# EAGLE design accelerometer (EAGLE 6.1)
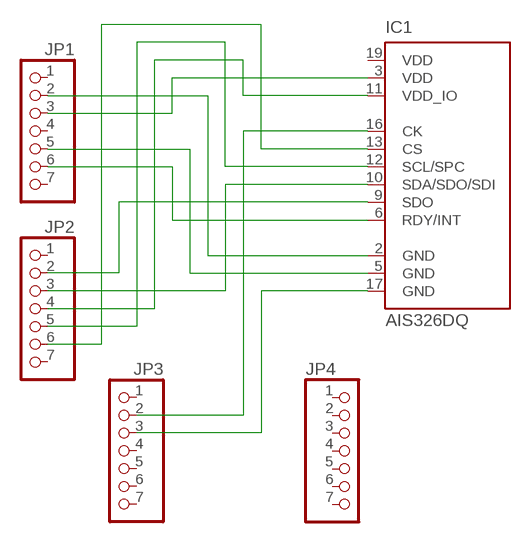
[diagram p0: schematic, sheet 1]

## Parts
IC1  AIS326DQ  [QFPN-28]
JP1  PINHD-1X7  [1X07]
JP2  PINHD-1X7  [1X07]
JP3  PINHD-1X7  [1X07]
JP4  PINHD-1X7  [1X07]

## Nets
N$1: IC1.2(GND) JP1.2
N$2: IC1.3(VDD) JP1.3
N$3: IC1.5(GND) JP1.5
N$4: IC1.6(RDY/INT) JP1.6
N$5: IC1.9(SDO) JP2.2
N$6: IC1.10(SDA/SDO/SDI) JP2.3
N$7: IC1.11(VDD_IO) JP2.4
N$8: IC1.12(SCL/SPC) JP2.5
N$9: IC1.13(CS) JP2.6
N$10: IC1.16(CK) JP3.2
N$11: IC1.17(GND) JP3.3
Unconnected: JP1.1 JP1.4 JP1.7 JP2.1 JP2.7 JP3.1 JP3.4 JP3.5 JP3.6 JP3.7 JP4.1 JP4.2 JP4.3 JP4.4 JP4.5 JP4.6 JP4.7

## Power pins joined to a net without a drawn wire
VDD: IC1.19(VDD)

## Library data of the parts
IC1 = cansat_jecnaci:AIS326DQ: MEMS INERTIAL SENSOR 3-Axis - ±2g/±6g Digital Output Low Voltage Linear Accelerometer Source: http://www.st.com; MF: Arrow Electronics; MPN: AIS326DQ; OC_FARNELL: 1220909; OC_NEWARK: 89K0642
JP1-JP4 = pinhead:PINHD-1X7: PIN HEADER

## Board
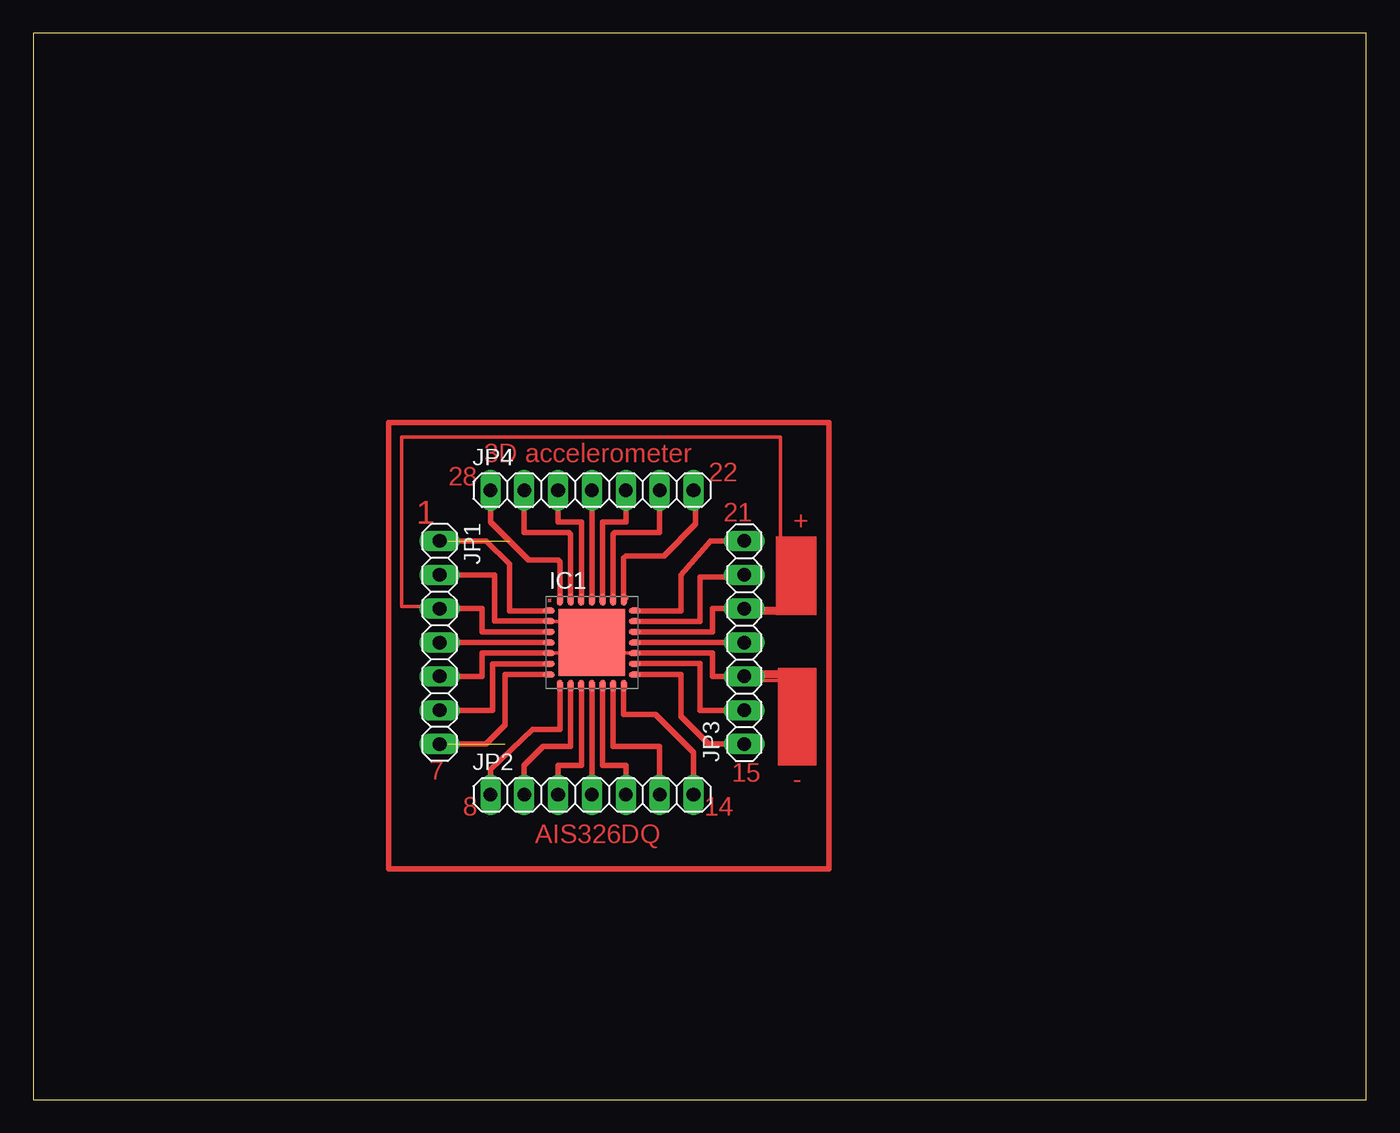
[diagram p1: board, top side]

Size 100 x 80 mm. Coordinates in mm from the lower left corner, seen from the top.
Outline: 0,0 100,0 100,80 0,80 0,0
Copper layers (1*16): Top 0.035mm / dielectric 1.5mm / Bottom 0.035mm
Design rules: minimum track width 10mil, minimum drill 24mil, track to track 8mil, track to pad 8mil, pad to pad 8mil, via to via 8mil, smd to smd 8mil, copper to edge 40mil, drill to drill 8mil, minimum pad ring 10mil, minimum via ring 8mil, stop-mask expansion 4mil, vias tented up to drill 0mil, thermal gap 10mil

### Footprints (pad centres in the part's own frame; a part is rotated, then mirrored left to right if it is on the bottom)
QFPN-28 = smd 0.9 x 0.45: 1 -3.225,2.4; 2 -3.225,1.6; 3 -3.225,0.8; 4 -3.225,0; 5 -3.225,-0.8; 6 -3.225,-1.6; 7 -3.225,-2.4; 15 3.225,-2.4; 16 3.225,-1.6; 17 3.225,-0.8; 18 3.225,0; 19 3.225,0.8; 20 3.225,1.6; 21 3.225,2.4 | smd 0.45 x 0.9: 8 -2.4,-3.225; 9 -1.6,-3.225; 10 -0.8,-3.225; 11 0,-3.225; 12 0.8,-3.225; 13 1.6,-3.225; 14 2.4,-3.225; 22 2.4,3.225; 23 1.6,3.225; 24 0.8,3.225; 25 0,3.225; 26 -0.8,3.225; 27 -1.6,3.225; 28 -2.4,3.225 | smd 5 x 5: TH 0,0
1X07 = drill 1.016 long: 1 -7.62,0; 2 -5.08,0; 3 -2.54,0; 4 0,0; 5 2.54,0; 6 5.08,0; 7 7.62,0

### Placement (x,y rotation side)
IC1  41.91,34.29 0 top
JP1  30.48,34.29 270 top
JP2  41.91,22.86 0 top
JP3  53.34,34.29 90 top
JP4  41.91,45.72 0 top

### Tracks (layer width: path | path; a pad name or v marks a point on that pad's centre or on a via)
N$1
  Top 0.406: IC1.2 34.61,35.89 34.61,39.37 JP1.2
N$2
  Top 0.406: IC1.3 33.66,35.09 33.66,36.83 JP1.3
N$3
  Top 0.406: IC1.5 33.66,33.49 33.66,31.75 JP1.5
N$4
  Top 0.406: IC1.6 34.45,32.69 34.45,29.21 JP1.6
N$5
  Top 0.406: IC1.9 40.32,31.07 40.32,26.51 38.26,26.51 36.83,25.08 JP2.2
N$6
  Top 0.406: IC1.10 41.12,25.08 39.37,25.08 JP2.3
N$7
  Top 0.406: IC1.11 JP2.4
N$8
  Top 0.406: IC1.12 42.7,25.08 44.45,25.08 JP2.5
N$9
  Top 0.406: IC1.13 43.5,31.07 43.5,26.51 46.99,26.51 JP2.6
N$10
  Top 0.406: IC1.16 45.15,32.7 50.01,32.7 50.01,29.21 JP3.2
N$11
  Top 0.406: IC1.17 50.96,33.5 50.96,31.75 JP3.3
N$12
  Top 0.406: 26.67,50.8 26.67,17.3 59.69,17.3 59.69,50.8 26.67,50.8
N$13
  Top 0.406: 31.11,34.29 38.58,34.29
N$14  (2 unrouted)
  Top 0.406: 38.42,31.91 35.4,31.91 35.4,28.1 33.97,26.67 31.75,26.67
N$15  (2 unrouted)
  Top 0.406: 38.73,36.67 35.72,36.67 35.72,40.16 33.97,41.91 30.48,41.91
N$16
  Top 0.406: 39.53,30.8 39.53,27.78 37.47,27.78 34.29,24.77 34.29,23.65
N$17
  Top 0.406: 45.4,34.29 52.39,34.29
N$18
  Top 0.406: 45.4,31.91 48.58,31.91 48.58,28.73 50.64,26.67 52.39,26.67
N$19
  Top 0.406: 44.29,30.8 44.29,28.89 46.67,28.89 49.53,26.04 49.53,23.81
N$20
  Top 0.406: 45.4,35.08 50.96,35.08 50.96,36.83 52.39,36.83
N$21
  Top 0.406: 45.24,35.88 50.01,35.88 50.01,39.21 52.39,39.21
N$22
  Top 0.406: 45.4,36.67 48.58,36.67 48.58,39.37 50.8,41.91 52.23,41.91
N$23
  Top 0.406: 41.91,37.62 41.91,44.77
N$24
  Top 0.406: 42.7,37.78 42.7,43.34 44.45,43.34 44.45,44.77
N$25
  Top 0.406: 43.5,37.78 43.5,42.39 43.66,42.55 46.99,42.55 46.99,44.61
N$26
  Top 0.406: 44.45,37.62 44.29,37.78 44.29,40.64 44.45,40.8 47.31,40.8 49.69,43.18 49.69,44.61
N$27
  Top 0.406: 41.12,37.62 41.12,43.34 39.37,43.34 39.37,44.77
N$28
  Top 0.406: 40.32,37.62 40.32,42.39 40.16,42.55 36.83,42.55 36.83,44.93
N$29
  Top 0.406: 39.53,37.78 39.53,40.32 39.37,40.48 37.15,40.48 34.29,43.34 34.29,44.61
N$30
  Top 0.254: 44.93,33.5 44.13,33.5
N$31
  Top 0.254: 38.89,35.88 39.69,35.88
N$32
  Top 0.254: 38.89,33.5 39.69,33.5
N$33
  Top 0.254: 29.53,36.99 27.62,36.99 27.62,49.69 56.04,49.69 56.04,36.83 54.13,36.83
N$34
  Top 0.254: 54.29,31.75 54.61,31.75 | 56.52,31.59 56.52,31.75 54.61,31.75 | 54.61,31.75 54.61,31.43 56.36,31.43
N$35
  Top 0.254: 55.88,36.67 56.04,36.67 | 54.45,36.67 54.61,36.67 | 54.61,36.67 55.88,36.67 | 55.88,36.67 55.88,36.51 54.61,36.51 54.61,36.67
N$36
  Top 0.254: 54.61,32.07 56.2,32.07
N$37
  Top 0.254: 54.77,31.91 56.2,31.91
(copper drawn outside any net)
  shapes: Top area x3

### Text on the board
Top: 3D accelerometer | 28 | 22 | 1 | 21 | + | 7 | 15 | - | 8 | 14 | AIS326DQ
